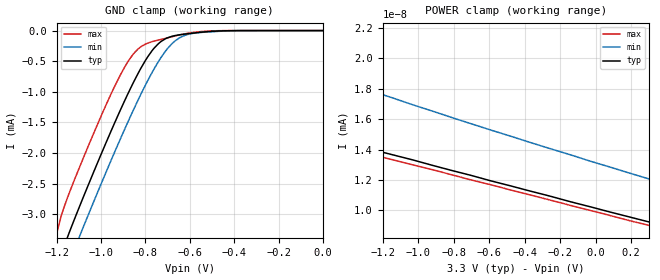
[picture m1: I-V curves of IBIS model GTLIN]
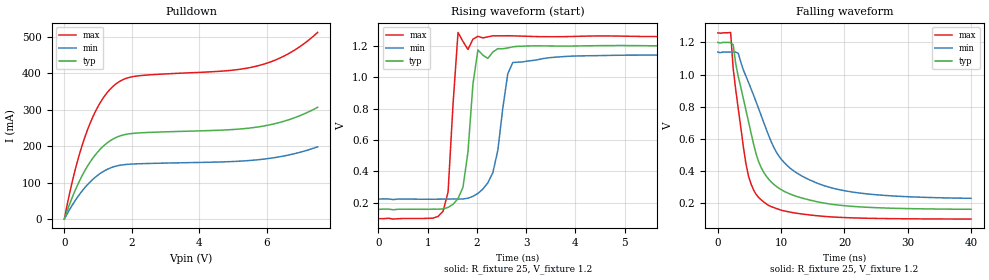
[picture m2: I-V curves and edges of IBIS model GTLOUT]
[IBIS Ver]   3.2
[Comment Char]   |_char
[File name]   gtl2034.ibs
[File Rev]   0
[Date]   May 2, 2006 1:57:42 PM
[Source]
[Notes]
[Disclaimer]
* Specialty Logic Products for Philips Semiconductors. Tempe, AZ
* K.Williams
*  Property of Philips Semiconductors *
*  Unauthorized reproduction and/or distribution is strictly *
*  prohibited.  (C) Copyright 2005 Philips Semiconductors. *
*  All rights reserved. *
*  PLEASE BE AWARE THAT IN THE ABSENCE OF A SIGNED, WRITTEN AGREEMENT *
*  TO THE CONTRARY, PHILIPS SEMICONDUCTORS (COMPANY) IS PROVIDING THE *
*  SPICE MODELS "AS IS" AND WITHOUT ANY WARRANTY, EXPRESSED OR IMPLIED.  *
*  Further, COMPANY assumes no liability for: 1) the accuracy of the *
*  SPICE models provided to your company; 2) the proper functioning of *
*  these SPICE models in your design or for any resulting applications;  *
*  or 3) infringement of patents, copyrights or intellectual property *
*  rights resulting from your use of these SPICE models. *
*  COMPANY provides SPICE models as a service to our customers.  You and *
*  your company shall not distribute, convey, sell or give these models  *
*  to anyone else without receiving prior written permission from *
*  COMPANY. *
*  COMPANY reserves the right to make changes to its products or to *
*  discontinue any semiconductor product or service without notice and *
*  advises its customers to obtain the latest version of relevant *
*  information to verify, before placing orders, that the information *
*  being relied on is current. *
*  Please be aware that your receipt and subsequent use of the SPICE *
*  information provided shall serve as acceptance of the terms and *
*  conditions of this agreement.  If you do not accept these terms, *
*  you should return the SPICE model and any other accompanying *
*  information immediately. *
[Copyright]
[Component]   GTL2034
Si_location Pin
Timing_location Pin
[Manufacturer]   Philips Semiconductor
[Package]
R_pkg   34.6m   28.0m   44.6m
L_pkg   2.04n   1.36n   2.32n
C_pkg   0.37pf   0.30pf   0.44pf
[Pin] signal_name   model_name
1   NC   NC
2   Bo0   GTLOUT
3   Bo1   GTLOUT
4   VREF   POWER
5   Bo2   GTLOUT
6   Bo3   GTLOUT
7   GND   GND
8   GND   GND
9   Bi3   GTLIN
10   Bi2   GTLIN
11   GND   GND
12   Bi1   GTLIN
13   Bi0   GTLIN
14   VCC   POWER
| Models and submodels in the file (2): GTLIN (Input), GTLOUT (Open_drain)
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[Model]   GTLIN
Model_type Input
Vinh=0.85
Vinl=0.75
C_comp   4.5p   4.5p   4.5p
[Model Spec]
[Temperature Range] 27   85   -40
[Voltage Range]   3.3   3.0   3.6
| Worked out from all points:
|   GND clamp passes 1 mA (typ) near -0.87 V on its own axis
|   POWER clamp passes 1 mA (typ) near -9.27 V on its own axis
[GND Clamp]
-1.5V     -1.188A    -662.4mA   -2.047A
-1.2V     -3.93mA    -4.411mA   -3.324mA
-1.14V    -3.272mA   -3.764mA   -2.627mA
-1.08V    -2.726mA   -3.214mA   -2.087mA
-920mV    -1.359mA   -1.832mA   -777.7uA
-860mV    -893.5uA   -1.346mA   -410.3uA
-820mV    -614.8uA   -1.039mA   -263.8uA
-730mV    -180.1uA   -442.6uA   -145.3uA
-680mV    -93.21uA   -213.4uA   -100.6uA
-620mV    -56.36uA   -75.67uA   -52.02uA
-420mV    -1.852uA   -4.796uA   -323.8nA
0V        0A         -3.307fA   0A
[POWER Clamp]
-10.7V    21.08A     19.98A     22.42A
-3.92V    22.57pA    30.75pA    21.66pA
-3.81V    22.2pA     30.1pA     21.34pA
-3.59V    21.46pA    28.82pA    20.69pA
-3.37V    20.72pA    27.57pA    19.98pA
-2.81V    18.93pA    24.67pA    18.33pA
-2.7V     18.53pA    24.13pA    18.02pA
-2.14V    16.77pA    21.5pA     16.33pA
-1.59V    15.05pA    19.16pA    14.68pA
-1.03V    13.32pA    16.94pA    12.99pA
-370mV    11.27pA    14.47pA    11.01pA
300mV     9.237pA    12.07pA    9.01pA
[Model]   GTLOUT
Model_type Open_drain
Vref=1.2
Vmeas=0.8
Rref=25
C_comp   5.5p   5.5p   5.5p
[Model Spec]
[Temperature Range] 27   85   -40
[Voltage Range]   3.3   3.0   3.6
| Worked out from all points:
|   slope of the pulldown table from 0 to 0.495 V, typ, clamps not added: 4.37 ohm
|   falling waveform, R_fixture 25, V_fixture 1.2: 20-80 % time 4.43ns typ, 6.83ns min, 2.68ns max; typ from 1.2 V to 0.161 V
|   rising waveform, R_fixture 25, V_fixture 1.2: 20-80 % time 188ps typ, 263ps min, 134ps max; typ from 0.159 V to 1.2 V
[Pulldown]
0V        -5.986uA   -6.235uA   -6.613uA
300mV     74.39mA    47.83mA    127.9mA
450mV     105.1mA    67.92mA    179.2mA
680mV     144.5mA    93.97mA    243.7mA
1.06V     191.7mA    125.1mA    319.4mA
1.29V     210.7mA    137.4mA    349.7mA
1.52V     223.5mA    145.1mA    370.6mA
2.12V     236mA      151.5mA    392.5mA
4.77V     244.7mA    157.2mA    407mA
5.76V     253.3mA    163.1mA    421.6mA
6.67V     273.5mA    176.5mA    455.8mA
7.5V      306.9mA    198.3mA    512.5mA
[Falling Waveform]
R_fixture=25
C_fixture=0
V_fixture=1.2
V_fixture_min=1.14
V_fixture_max=1.26
0s        1.2V       1.14V      1.26V
2.02ns    1.199V     1.14V      1.262V
2.424ns   1.186V     1.14V      1.038V
3.232ns   986.3mV    1.132V     784.8mV
4.444ns   777.4mV    989.4mV    443mV
5.657ns   566mV      870.2mV    279.8mV
7.677ns   365.9mV    656.6mV    194mV
10.91ns   264.5mV    434.9mV    147.3mV
16.57ns   201mV      310.9mV    117.4mV
40ns      160.8mV    229.1mV    100mV
[Rising Waveform]
R_fixture=25
V_fixture=1.2
V_fixture_min=1.14
V_fixture_max=1.26
0s        159mV      223.8mV    99.48mV
1.313ns   161.8mV    224mV      147.6mV
1.414ns   171.3mV    224.4mV    269mV
1.616ns   227.7mV    224.7mV    1.284V
1.818ns   525.1mV    230mV      1.176V
1.919ns   957mV      241.7mV    1.242V
2.02ns    1.173V     260.4mV    1.26V
2.323ns   1.16V      392.5mV    1.263V
2.727ns   1.193V     1.093V     1.263V
10ns      1.2V       1.14V      1.26V
[Ramp]
R_load=25
dV/dt_r   6.246E-1/1.653E-10   5.782E-1/2.475E-10   6.633E-1/1.126E-10
dV/dt_f   6.236E-1/4.429E-9   5.748E-1/6.978E-9   6.630E-1/2.575E-9
|[End   GTLOUT
